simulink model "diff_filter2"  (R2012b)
settings: Solver=ode45  StartTime=0.0  StopTime=20  MaxStep=0.001  RelTol=1e-3
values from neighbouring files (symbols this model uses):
  dt1 = 0.01    [diff_filter_2.m]
  gama = 1e4    (= 10000)    [diff_filter_1.m]    (also in diff_filter_2.m)
  k = 10    [coulomb_10.m]    (also in coulomb_11.m; diff_filter_1.m = 250; diff_filter_2.m = 250; dry_friction_1.m = 2200)
  noise_g = 1    [diff_filter_2.m]
  noise_m = sqrt(varianz)    [diff_filter_2.m]
libraries: dsparch4 x1

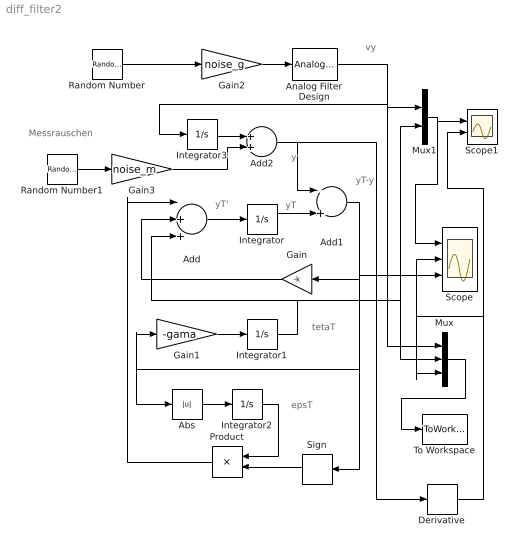
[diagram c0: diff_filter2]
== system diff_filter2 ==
  note: vy
  note: Messrauschen
  note: tetaT
  note: epsT
  note: yT-y
  note: y
  note: yT'
  note: yT
  Abs : Abs  ZeroCross=off
  Add : Sum  Inputs=-++
  Add1 : Sum  Inputs=-+
  Add2 : Sum
  Analog Filter Design : dsparch4/Analog Filter Design  method=Butterworth  filttype=Lowpass  N=4  Wlo=w_pass  Whi=80  Rp=2  Rs=40
  Derivative : Derivative
  Gain : Gain  Gain=-k
  Gain1 : Gain  Gain=-gama
  Gain2 : Gain  Gain=noise_g
  Gain3 : Gain  Gain=noise_m
  Integrator{,1..3} (4 alike) : Integrator
  Mux : Mux  Inputs=3
  Mux1 : Mux  Inputs=2
  Product : Product
  Random Number : RandomNumber  Seed=1305793  SampleTime=dt1
  Random Number1 : RandomNumber  Seed=13093  SampleTime=0
  Scope : Scope  NumInputPorts=3
  Scope1 : Scope  NumInputPorts=2
  Sign : Signum  ZeroCross=off
  To Workspace : ToWorkspace  VariableName=y  SampleTime=-1  SaveFormat=Structure With Time
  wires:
  Add/1 -> Integrator/1
  Integrator/1 -> Add1/2
  Gain/1 -> Add/2
  Gain1/1 -> Integrator1/1
  Abs/1 -> Integrator2/1
  Integrator2/1 -> Product/1
  Sign/1 -> Product/2
  Product/1 -> Add/1
  Integrator1/1 -> Add/3, Mux/2, Mux1/2
  Random Number/1 -> Gain2/1
  Add1/1 -> Scope/3, Sign/1, Abs/1, Gain1/1, Gain/1
  Mux/1 -> To Workspace/1
  Gain2/1 -> Analog Filter Design/1
  Mux1/1 -> Scope/1, Scope1/1
  Analog Filter Design/1 -> Mux/1, Integrator3/1, Mux1/1
  Integrator3/1 -> Add2/1
  Random Number1/1 -> Gain3/1
  Gain3/1 -> Add2/2
  Add2/1 -> Add1/1, Derivative/1
  Derivative/1 -> Scope/2, Mux/3, Scope1/2
